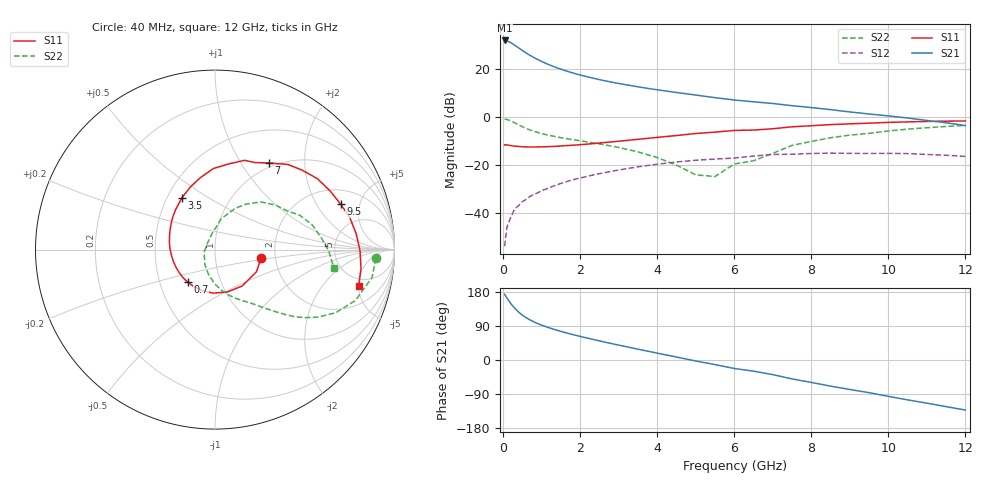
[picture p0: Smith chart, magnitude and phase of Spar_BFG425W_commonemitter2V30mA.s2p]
! Filename: 230bfg425.001
! BFG425W Field C1
! V1=8.711E-001V,V2=2.000E+000V, I1=4.441E-004A, I2=3.004E-002A
# GHz  S  MA  R 50
!  S11  S21  S12  S22
!Freq(GHz)  Mag  Ang  Mag  Ang  Mag  Ang  Mag  Ang
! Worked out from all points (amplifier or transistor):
!   44 points, 40 MHz to 12 GHz, reference 50 ohm
!   highest |S21| = 32.0 dB at 40 MHz (marker M1)
!   |S21| within 3 dB of that: start of sweep to 393.2 MHz
!   unconditionally stable (mu >= 1): start of sweep to 48.46 MHz; 1.007 GHz to end of sweep
!   at 700 MHz: K = 0.88, MSG = 29.5 dB, |S12| = -33.2 dB
!   at 2.4 GHz: K = 1.19, MAG = 17.4 dB, |S12| = -24.0 dB
!   at 12 GHz: K = 1.36, MAG = 2.9 dB, |S12| = -16.5 dB
!   lowest NFmin = 2.30 dB at 900 GHz
!   S11 on the Smith chart (normalised r, x): 40 MHz: 1.68, -0.17; 700 MHz: 0.69, -0.27; 3.5 GHz: 0.59, +0.39; 7 GHz: 0.94, +1.33; 9.5 GHz: 2.88, +3.28; 12 GHz: 3.90, -5.01
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0.04  0.261 -10.6  39.77 173.1  0.002 85.6  0.897 -3.0
0.1  0.262 -28.2  38.93 163.7  0.005 82.7  0.889 -10.0
0.2  0.253 -53.2  35.87 148.9  0.008 75.4  0.832 -19.9
0.3  0.246 -73.9  31.75 136.8  0.012 71.8  0.759 -27.6
0.4  0.243 -92.4  27.91 126.8  0.014 68.9  0.688 -33.1
0.5  0.239 -107.8  24.56 118.3  0.017 66.3  0.628 -37.1
0.6  0.237 -119.8  21.76 111.5  0.019 65.2  0.578 -40.2
0.7  0.237 -129.6  19.44 105.8  0.022 64.3  0.536 -42.5
0.9  0.237 -146.1  15.87 96.1  0.026 63.0  0.475 -46.3
1.2  0.241 -164.0  12.31 84.8  0.033 60.9  0.413 -50.8
1.7  0.254 174.1  8.859 70.0  0.046 56.7  0.348 -57.9
2.2  0.272 157.3  6.881 57.5  0.058 51.2  0.3 -65.9
2.8  0.301 140.2  5.391 43.7  0.073 43.6  0.248 -76.6
3.5  0.342 122.8  4.276 28.6  0.091 33.6  0.187 -91.4
4.5  0.41 101.3  3.255 7.9  0.115 18.2  0.099 -125.1
5.5  0.483 81.0  2.538 -12.1  0.132 2.3  0.057 134.3
6.5  0.534 65.2  2.079 -29.4  0.153 -10.5  0.122 87.7
7  0.568 58.2  1.917 -38.6  0.165 -18.4  0.174 79.0
8.5  0.694 34.7  1.426 -69.0  0.176 -47.2  0.369 46.0
9.5  0.744 20.0  1.157 -86.2  0.173 -63.6  0.455 28.4
10.5  0.791 6.6  0.953 -105.2  0.172 -81.8  0.558 14.5
12  0.826 -14.3  0.662 -132.0  0.15 -110.9  0.67 -8.7
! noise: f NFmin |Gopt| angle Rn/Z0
900  2.3  0.29  -166.5  0.19
2000  2.8  0.27  -150.8  0.25
